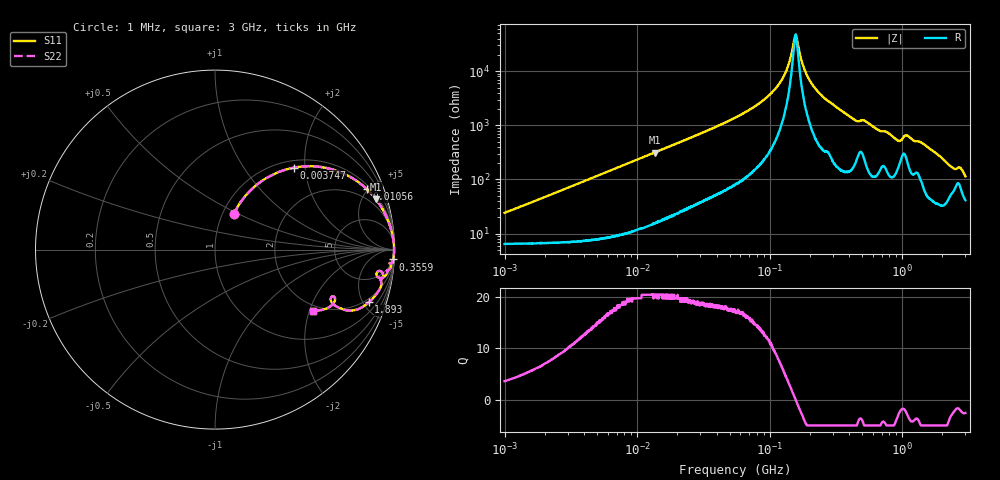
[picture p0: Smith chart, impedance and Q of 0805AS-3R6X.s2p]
!s-Parameter Generated by FASTRON Sdn. Bhd.
!FASTRON P/N : 0805AS-3R6X
!Keysight Technologies: E4991B_MY54100416_A.01.15
!Date: Mon Jun 15 12:58:53 2026
!Version  :Rev01  Mon Jun 15 12:58:53 2026
!Data & Calibration Information:
!Freq  S11  S21  S12  S22
!PortZ  Port1:50+j0  Port2:50+j0
!When reading reference impedance value at option line is always used.
! Remarks : This data is being provided solely for informational purposes.
# Hz S dB R 50
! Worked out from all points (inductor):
!   1601 points, 1 MHz to 3 GHz, reference 50 ohm
!   read as one part in series: L = 3.72 uH near 1.041 MHz
!   highest Q = 20.5 at 13.56 MHz (marker M1), where L = 3.69 uH
!   self-resonance near 156.7 MHz
!   S11 on the Smith chart (normalised r, x): 1 MHz: 1.13, +0.46; 3.747 MHz: 1.14, +1.75; 10.56 MHz: 1.25, +4.91; 355.9 MHz: 4, -36; 1.893 GHz: 1.69, -5.51; 3 GHz: 1.83, -2.12
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1000000  -13.10 62.2  -0.75 -12.4  -0.75 -12.4  -13.10 62.2
1965088  -7.98 58.5  -1.30 -23.3  -1.30 -23.3  -7.98 58.5
3747356  -3.96 46.1  -2.81 -39.2  -2.81 -39.2  -3.96 46.1
3804036  -3.89 45.8  -2.87 -39.6  -2.87 -39.6  -3.89 45.8
1.05579e7  -0.81 21.7  -8.62 -65.4  -8.62 -65.4  -0.81 21.7
1.355931e7  -0.54 17.3  -10.50 -69.9  -10.50 -69.9  -0.54 17.3
1.447069e7  -0.48 16.3  -11.00 -70.9  -11.00 -70.9  -0.48 16.3
5.504702e7  -0.06 4.1  -22.90 -82.6  -22.90 -82.6  -0.06 4.1
8.550185e7  -0.03 2.1  -28.50 -83.7  -28.50 -83.7  -0.03 2.1
1.142934e8  -0.02 1.1  -34.50 -82.1  -34.50 -82.1  -0.02 1.1
1.348146e8  -0.02 0.5  -40.70 -75.8  -40.70 -75.8  -0.02 0.5
1.566509e8  -0.02 0.0  -53.20 -4.5  -53.20 -4.5  -0.02 0.0
1.614254e8  -0.02 -0.1  -51.50 35.6  -51.50 35.6  -0.02 -0.1
1.820241e8  -0.02 -0.5  -41.00 75.1  -41.00 75.1  -0.02 -0.5
2.083556e8  -0.02 -1.0  -35.30 80.9  -35.30 80.9  -0.02 -1.0
2.570867e8  -0.03 -1.8  -30.20 82.2  -30.20 82.2  -0.03 -1.8
3.55908e8  -0.05 -3.2  -25.10 82.3  -25.10 82.3  -0.05 -3.2
7.925923e8  -0.28 -7.7  -17.30 72.5  -17.30 72.5  -0.28 -7.7
9.349007e8  -0.64 -9.8  -15.00 61.7  -15.00 61.7  -0.64 -9.8
1.091779e9  -0.51 -7.9  -16.70 62.9  -16.70 62.9  -0.51 -7.9
1.893158e9  -0.86 -18.9  -9.75 64.0  -9.75 64.0  -0.86 -18.9
3e9  -3.82 -31.8  -4.96 36.9  -4.96 36.9  -3.82 -31.8
